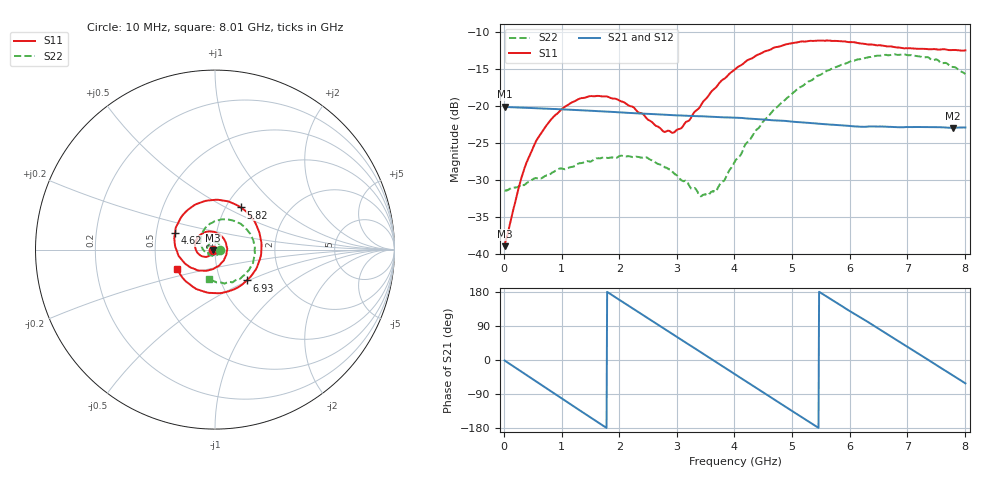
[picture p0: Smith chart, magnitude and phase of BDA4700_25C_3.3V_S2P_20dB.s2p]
!Agilent Technologies,E5071B,MY42404982,A.09.10
!Date: Mon Oct 20 18:11:27 2025
!Data & Calibration Information:
!Freq	S11:SOLT2(ON)	S21:SOLT2(ON)	S12:SOLT2(ON)	S22:SOLT2(ON)
# Hz S RI R 50
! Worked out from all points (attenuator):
!   801 points, 10 MHz to 8.01 GHz, reference 50 ohm
!   highest |S21| = -20.08 dB at 10 MHz (marker M1); lowest = -22.9 dB at 7.8 GHz (marker M2)
!   lowest |S11| = -38.9 dB at 10 MHz (marker M3), VSWR 1.02, Z = 48.9 - j0.164 ohm
!   |S11| at or under -10 dB: start of sweep to end of sweep
!   |S22| runs from -32.2 to -13.0 dB; largest |S21 - S12| = 0.0011
!   S11 on the Smith chart (normalised r, x): 10 MHz: 0.98, -0.00; 4.62 GHz: 0.63, +0.12; 5.82 GHz: 1.17, +0.60; 6.93 GHz: 1.33, -0.49; 8.01 GHz: 0.64, -0.14
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1e7  -0.0112 -0.00168  0.0991 -0.00213  0.0991 -0.00223  0.0269 -0.000826
3.2e8  -0.022 -0.0267  0.082 -0.0531  0.0821 -0.0531  0.0239 -0.0167
5.6e8  -0.043 -0.0396  0.0526 -0.0813  0.0526 -0.0814  0.0153 -0.0288
8.7e8  -0.0782 -0.0347  0.00274 -0.0957  0.00278 -0.0957  -0.0065 -0.0356
1.35e9  -0.1115 0.0212  -0.068 -0.0646  -0.068 -0.0647  -0.0372 -0.0179
1.96e9  -0.0532 0.0979  -0.087 0.0269  -0.0871 0.0268  -0.0349 0.0282
2.45e9  0.0322 0.0787  -0.0371 0.0807  -0.0372 0.0807  -0.00173 0.0453
2.68e9  0.0599 0.0408  -0.00333 0.0879  -0.00352 0.0879  0.0147 0.0378
2.96e9  0.064 -0.0188  0.0367 0.0786  0.0367 0.0785  0.0273 0.0218
3.43e9  -0.00203 -0.1034  0.0807 0.028  0.0808 0.0281  0.0198 -0.0147
3.69e9  -0.0682 -0.1172  0.084 -0.00911  0.084 -0.00934  0.000478 -0.0268
4.01e9  -0.1547 -0.0868  0.0662 -0.051  0.0664 -0.0509  -0.0328 -0.0267
4.62e9  -0.2219 0.0931  -0.0105 -0.08  -0.0103 -0.08  -0.0796 0.0381
4.95e9  -0.1725 0.2007  -0.0504 -0.0609  -0.0502 -0.0612  -0.0707 0.093
5.35e9  -0.0384 0.2736  -0.0753 -0.0154  -0.0752 -0.0158  -0.0155 0.1494
5.82e9  0.1438 0.235  -0.0622 0.0409  -0.062 0.041  0.0903 0.1645
6.25e9  0.2476 0.0935  -0.0207 0.0695  -0.0197 0.0697  0.1829 0.1049
6.68e9  0.239 -0.0856  0.0301 0.0659  0.0303 0.066  0.2215 -0.00297
6.93e9  0.1774 -0.1716  0.0535 0.0482  0.0537 0.0479  0.2127 -0.0732
7.35e9  0.0148 -0.2431  0.0722 0.00223  0.0723 0.00221  0.1391 -0.1634
7.8e9  -0.1633 -0.176  0.0537 -0.047  0.0537 -0.0472  0.0159 -0.1834
8.01e9  -0.214 -0.1057  0.0341 -0.0632  0.0343 -0.063  -0.0339 -0.1616
